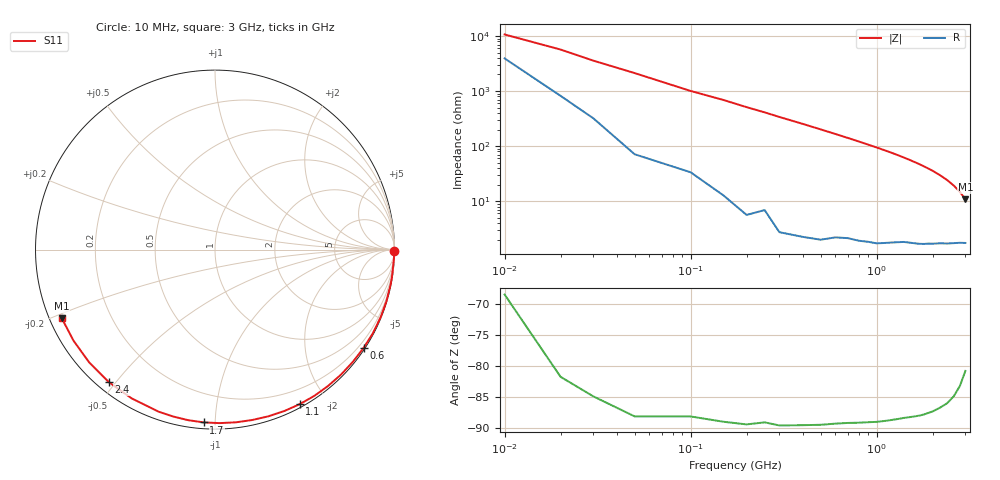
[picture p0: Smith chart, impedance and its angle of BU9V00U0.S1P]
! SIEMENS Small Signal Semiconductors
! BB833
! Si Tuning Diode in SOD323
! VR = 9 V
! S-Parameters:  April  1996
# GHz  S  MA  R  50
!  f  S11
! GHz  MAG  ANG
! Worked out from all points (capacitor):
!   31 points, 10 MHz to 3 GHz, reference 50 ohm
!   read as one part to ground: C = 1.49 pF near 10 MHz
!   lowest |Z| = 10.8 ohm at 3 GHz (marker M1)
!   S11 on the Smith chart (normalised r, x): 10 MHz: open; 600 MHz: 0.04, -3.32; 1.1 GHz: 0.03, -1.69; 1.7 GHz: 0.03, -0.94; 2.4 GHz: 0.03, -0.48; 3 GHz: 0.03, -0.21
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0.01  0.9966 -0.5
0.05  0.9984 -2.7
0.1  0.9967 -5.7
0.15  0.9973 -8.3
0.2  0.9979 -11.2
0.3  0.9977 -16.8
0.4  0.9966 -22.3
0.5  0.9954 -27.9
0.6  0.9927 -33.5
0.7  0.9905 -39.1
0.8  0.989 -44.7
0.9  0.9869 -50.3
1  0.9851 -55.8
1.1  0.9821 -61.3
1.2  0.9788 -66.7
1.3  0.9753 -72.2
1.4  0.9718 -77.7
1.5  0.9694 -83.1
1.6  0.9671 -88.5
1.7  0.9649 -93.7
1.8  0.9621 -98.9
1.9  0.9588 -104.0
2  0.9561 -109.1
2.2  0.9502 -119.2
2.4  0.9461 -128.8
2.6  0.9414 -138.2
2.8  0.9375 -147.2
3  0.9355 -155.8
